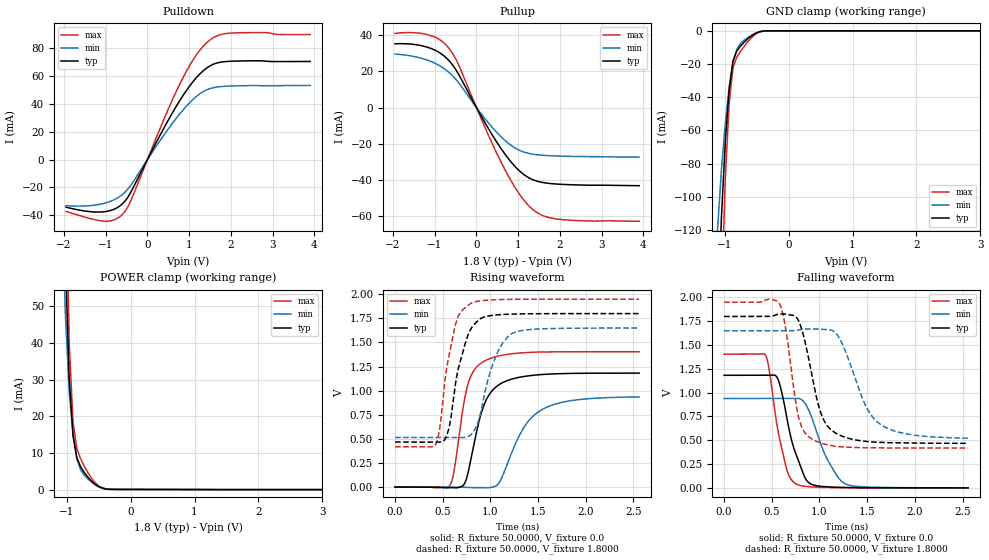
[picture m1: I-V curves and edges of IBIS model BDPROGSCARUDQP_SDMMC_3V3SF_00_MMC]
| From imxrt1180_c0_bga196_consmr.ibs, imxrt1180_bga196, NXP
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[Model]  BDPROGSCARUDQP_SDMMC_3V3SF_00_MMC
|   Model BDPROGSCARUDQP_SDMMC_3V3SF_00_MMC
| This model was characterised for following simulation conditions:
| External (pad) voltage:
|   - Typ: 1.8V,   - Min: 1.65V,   - Max: 1.95V
| Library cells for typ/min/max conditions are connected as defined below:
|  IO - External Pad
|  A - Core Input
|  EN - Output Buffer Enable
|  ASRCN3V3[0] - gnde REFH3V3 gnde
|  ASRCN3V3[1] - REFH3V3 gnde gnde
|  ASRCN3V3[2] - gnde
|  ASRCN3V3[3] - gnde REFH3V3 gnde
|  ASRCP3V3[0] - vdde3v3 vdde3v3 REFL3V3
|  ASRCP3V3[1] - vdde3v3 REFL3V3 vdde3v3
|  ASRCP3V3[2] - REFL3V3 vdde3v3 vdde3v3
|  ASRCP3V3[3] - vdde3v3 REFL3V3 vdde3v3
|  IOGC - NC
|  PDRV - gnd
|  PSW - gnd
|  REFH3V3 - REFH3V3
|  REFL3V3 - REFL3V3
|  ZI - NC
|  gnd - gnd
|  gnde - gnde
|  vdd - vdd
|  vdde3v3 - vdde3v3
| All other pins connected to ground
Model_type I/O
Polarity   Non-Inverting
Enable   Active-Low
Vinl =   0.5775V
Vinh =   1.2675V
Vmeas =  0.9000V
Cref =   30.0000pF
Rref =   1.0000M
Vref =   1.8000V
C_comp   2.2202pF   2.2062pF   2.2431pF
|C_comp_pullup   1.1647pF   1.1333pF   1.1988pF
|C_comp_pulldown   0.7687pF   0.7945pF   0.7484pF
[Model Spec]
| variable   typ   min   max
Vinh   1.1700V   1.0725V   1.2675V
Vinl   0.6300V   0.5775V   0.6825V
[Temperature Range]   25.0000   0.1050k   -20.0000
[Voltage Range]   1.8000V   1.6500V   1.9500V
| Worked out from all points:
|   slope of the pulldown table from 0 to 0.27 V, typ, clamps not added: 17.2 ohm
|   slope of the pullup table from 0 to 0.27 V, typ, clamps not added: 24.6 ohm
|   GND clamp passes 1 mA (typ) near -0.49 V on its own axis
|   POWER clamp passes 1 mA (typ) near -0.52 V on its own axis
|   rising waveform, R_fixture 50.0000, V_fixture 0.0: 20-80 % time 193ps typ, 305ps min, 146ps max; typ from 0 V to 1.18 V
|   rising waveform, R_fixture 50.0000, V_fixture 1.8000: 20-80 % time 161ps typ, 197ps min, 139ps max; typ from 0.468 V to 1.8 V
|   falling waveform, R_fixture 50.0000, V_fixture 0.0: 20-80 % time 180ps typ, 232ps min, 145ps max; typ from 1.18 V to 0 V
|   falling waveform, R_fixture 50.0000, V_fixture 1.8000: 20-80 % time 186ps typ, 278ps min, 135ps max; typ from 1.8 V to 0.468 V
[Pulldown]
|Voltage   I(typ)   I(min)   I(max)
-1.95V    -34.28mA   -33.13mA   -37.33mA
-990mV    -37.37mA   -31.06mA   -44.43mA
-750mV    -35.06mA   -28.17mA   -42.78mA
-570mV    -31.01mA   -24.41mA   -38.56mA
-390mV    -23.02mA   -18.13mA   -29.05mA
390mV     22.39mA    17.45mA    28.62mA
810mV     44.08mA    34.16mA    56.43mA
1.17V     58.87mA    45.33mA    75.23mA
1.53V     67.94mA    51.38mA    86.75mA
1.77V     70.2mA     52.57mA    90.08mA
2.07V     70.86mA    53.03mA    91.16mA
3.9V      70.64mA    53.39mA    89.99mA
[Pullup]
|Voltage   I(typ)   I(min)   I(max)
-1.95V    35.27mA    29.56mA    41.01mA
-1.14V    33.09mA    25.92mA    40.12mA
-900mV    30.57mA    23.38mA    37.83mA
-660mV    25.99mA    19.47mA    32.84mA
-420mV    18.1mA     13.5mA     23.25mA
180mV     -7.422mA   -5.453mA   -9.694mA
660mV     -25.01mA   -17.72mA   -33.32mA
1.02V     -34.83mA   -23.55mA   -47.59mA
1.38V     -40.19mA   -25.93mA   -56.98mA
1.68V     -41.81mA   -26.57mA   -60.53mA
2.04V     -42.5mA    -26.9mA    -62mA
3.9V      -43.26mA   -27.44mA   -62.96mA
[GND_clamp]
|Voltage   I(typ)   I(min)   I(max)
-1.95V    -1.789A    -1.03A     -2.95A
-1.11V    -176.3mA   -119.2mA   -277.9mA
-1.05V    -112.3mA   -83.66mA   -163.2mA
-990mV    -66.82mA   -55.78mA   -89.16mA
-930mV    -35.58mA   -34.18mA   -43.87mA
-870mV    -18.33mA   -19.06mA   -22.3mA
-810mV    -12.12mA   -11.08mA   -15.87mA
-750mV    -9.12mA    -7.575mA   -12.28mA
-570mV    -2.717mA   -2.477mA   -3.751mA
-450mV    -466.5uA   -625uA     -610.9uA
-330mV    -31.46uA   -57.07uA   -36.76uA
3.9V      0A         0A         0A
[POWER_clamp]
|Voltage   I(typ)   I(min)   I(max)
-1.95V    1.733A     983.2mA    2.899A
-1.08V    123mA      81.32mA    204.7mA
-1.02V    63.28mA    48.12mA    95.46mA
-960mV    30.45mA    27.05mA    40.34mA
-900mV    14.89mA    14.83mA    18.42mA
-840mV    8.668mA    8.37mA     11.21mA
-780mV    6.192mA    5.372mA    8.379mA
-720mV    4.573mA    3.84mA     6.25mA
-600mV    2.107mA    1.918mA    2.859mA
-480mV    625.6uA    714.7uA    800.1uA
-300mV    67.29uA    79.42uA    85.49uA
3.9V      0A         0A         0A
[Ramp]
| variable   typ   min   max
dV/dt_r  0.7089/0.1931n   0.5611/0.3045n   0.8421/0.1462n
dV/dt_f  0.7989/0.1861n   0.6768/0.2781n   0.9185/0.1351n
R_load = 50.0000
[Rising Waveform]
R_fixture= 50.0000
V_fixture= 0.0
V_fixture_min= 0.0
V_fixture_max= 0.0
|time   V(typ)   V(min)   V(max)
0s        129.7uV    113.6uV    158.4uV
576.2ps   -6.009mV   145.3uV    20.45mV
621.3ps   -6.808mV   289.2uV    181.7mV
715.1ps   18.1mV     -1.479mV   832.9mV
760.5ps   129.7mV    -3.968mV   1.054V
932.1ps   849.9mV    -6.889mV   1.304V
1.086ns   1.059V     37.64mV    1.359V
1.345ns   1.146V     609.9mV    1.393V
1.548ns   1.168V     807.5mV    1.401V
2.56ns    1.182V     935.3mV    1.404V
[Rising Waveform]
R_fixture= 50.0000
V_fixture= 1.8000
V_fixture_min= 1.6500
V_fixture_max= 1.9500
|time   V(typ)   V(min)   V(max)
0s        467.5mV    514.6mV    418.4mV
425.5ps   467.5mV    514.7mV    441.8mV
468.5ps   466.4mV    514.7mV    609.9mV
546.4ps   548.2mV    514.7mV    1.266V
628.7ps   1.036V     514.7mV    1.669V
793.2ps   1.637V     540.5mV    1.903V
875.2ps   1.732V     688.7mV    1.928V
1.055ns   1.784V     1.352V     1.943V
1.223ns   1.794V     1.591V     1.947V
2.56ns    1.799V     1.649V     1.949V
[Falling Waveform]
R_fixture= 50.0000
V_fixture= 0.0
V_fixture_min= 0.0
V_fixture_max= 0.0
|time   V(typ)   V(min)   V(max)
0s        1.182V     938.1mV    1.404V
435.3ps   1.181V     938.3mV    1.393V
474.6ps   1.182V     938.4mV    1.231V
567.9ps   1.134V     938.2mV    584.5mV
666.1ps   693.1mV    938.1mV    163.3mV
750.2ps   363.6mV    939.6mV    43.38mV
894.3ps   50.18mV    800.8mV    11.66mV
1.075ns   11mV       314.7mV    4.057mV
1.273ns   3.921mV    40.73mV    1.556mV
2.56ns    148.6uV    397.5uV    160.9uV
[Falling Waveform]
R_fixture= 50.0000
V_fixture= 1.8000
V_fixture_min= 1.6500
V_fixture_max= 1.9500
|time   V(typ)   V(min)   V(max)
0s        1.799V     1.649V     1.949V
573.8ps   1.823V     1.649V     1.947V
637.3ps   1.823V     1.649V     1.725V
778.8ps   1.759V     1.657V     753mV
920.9ps   1.184V     1.669V     512.7mV
1.036ns   733.2mV    1.664V     464.3mV
1.221ns   549.4mV    1.55V      431.2mV
1.478ns   488.7mV    875.1mV    421.5mV
1.637ns   477.7mV    668mV      419.7mV
2.56ns    467.7mV    521.3mV    418.3mV
